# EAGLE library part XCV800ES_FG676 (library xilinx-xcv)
xcv800es_fg676 edit this description Auto generated by make-symbol-device-package-bsdl.ulp Rev. 26 Source: xcv800es_fg676.bsd
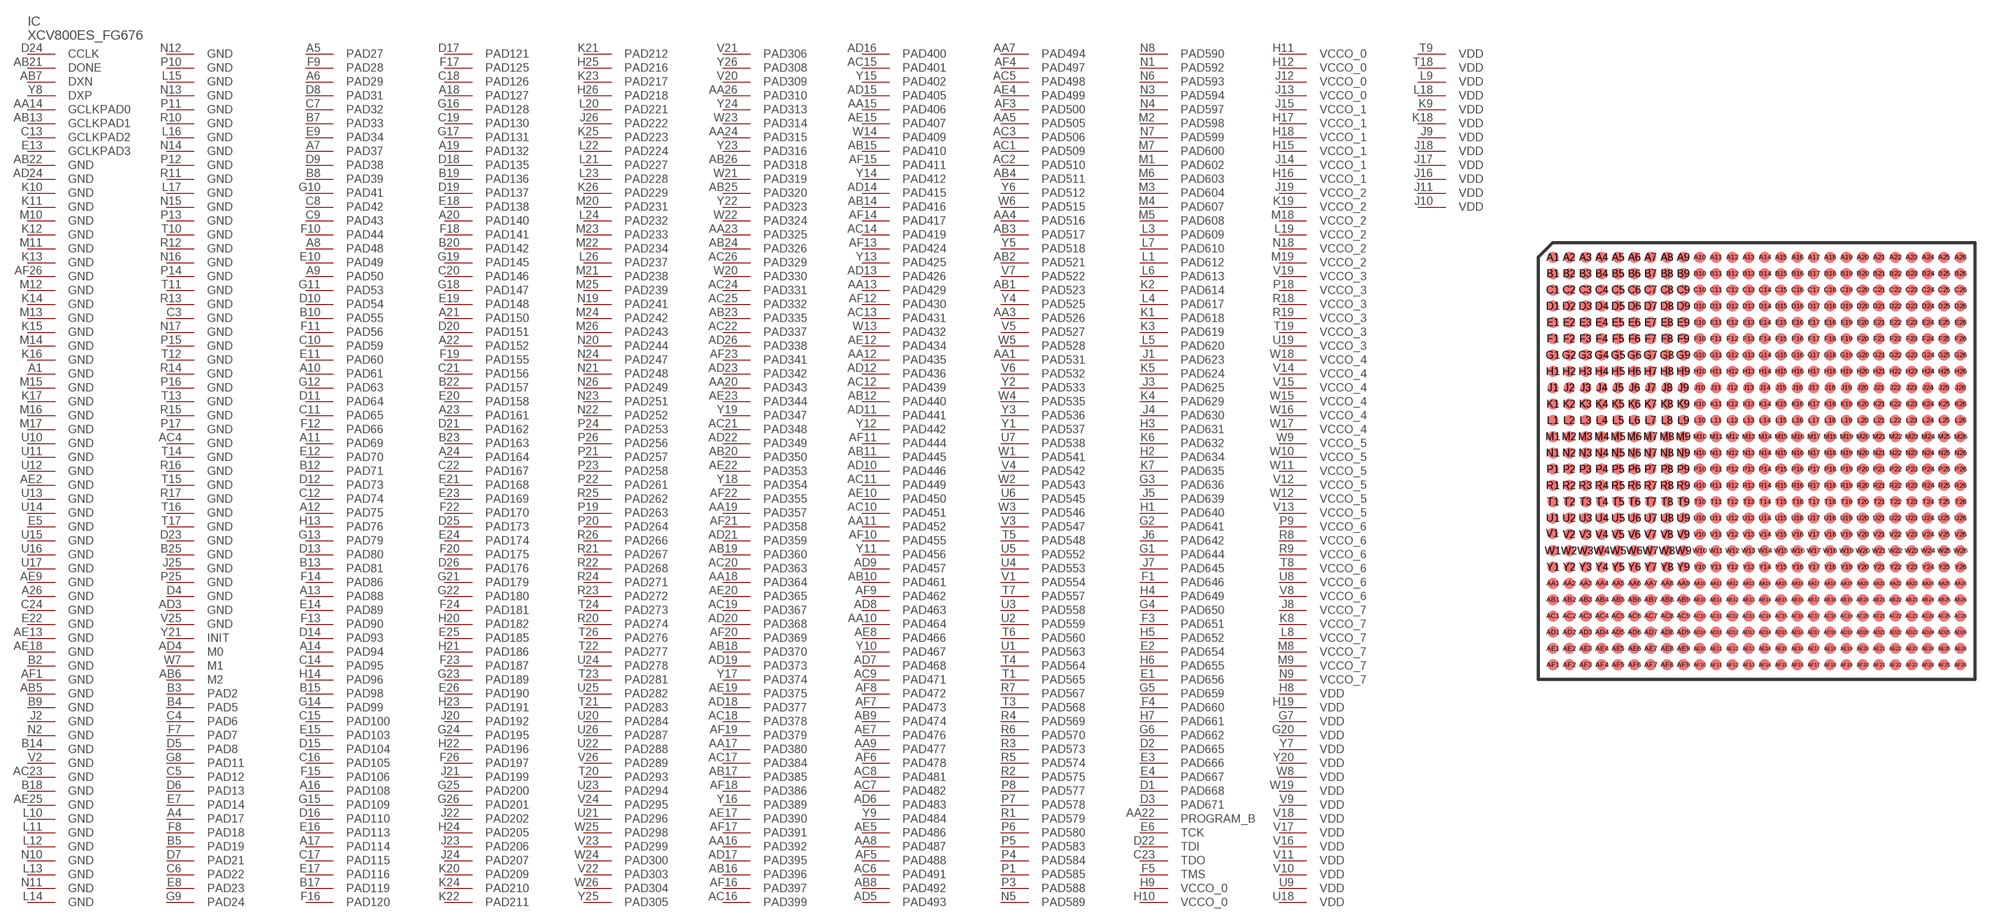
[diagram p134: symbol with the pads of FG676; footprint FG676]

Designator prefix IC

## XCV800ES_FG676 (OC_FARNELL: unknown; OC_NEWARK: unknown)  [FG676]
A1  GND  pwr
A4  PAD17
A5  PAD27
A6  PAD29
A7  PAD37
A8  PAD48
A9  PAD50
A10  PAD61
A11  PAD69
A12  PAD75
A13  PAD88
A14  PAD94
A16  PAD108
A17  PAD114
A18  PAD127
A19  PAD132
A20  PAD140
A21  PAD150
A22  PAD152
A23  PAD161
A24  PAD164
A26  GND  pwr
AA1  PAD531
AA3  PAD526
AA4  PAD516
AA5  PAD505
AA7  PAD494
AA8  PAD487
AA9  PAD477
AA10  PAD464
AA11  PAD452
AA12  PAD435
AA13  PAD429
AA14  GCLKPAD0  in
AA15  PAD406
AA16  PAD392
AA17  PAD380
AA18  PAD364
AA19  PAD357
AA20  PAD343
AA22  PROGRAM_B  in
AA23  PAD325
AA24  PAD315
AA26  PAD310
AB1  PAD523
AB2  PAD521
AB3  PAD517
AB4  PAD511
AB5  GND  pwr
AB6  M2  in
AB7  DXN  pas
AB8  PAD492
AB9  PAD474
AB10  PAD461
AB11  PAD445
AB12  PAD440
AB13  GCLKPAD1  in
AB14  PAD416
AB15  PAD410
AB16  PAD396
AB17  PAD385
AB18  PAD370
AB19  PAD360
AB20  PAD350
AB21  DONE
AB22  GND  pwr
AB23  PAD335
AB24  PAD326
AB25  PAD320
AB26  PAD318
AC1  PAD509
AC2  PAD510
AC3  PAD506
AC4  GND  pwr
AC5  PAD498
AC6  PAD491
AC7  PAD482
AC8  PAD481
AC9  PAD471
AC10  PAD451
AC11  PAD449
AC12  PAD439
AC13  PAD431
AC14  PAD419
AC15  PAD401
AC16  PAD399
AC17  PAD384
AC18  PAD378
AC19  PAD367
AC20  PAD363
AC21  PAD348
AC22  PAD337
AC23  GND  pwr
AC24  PAD331
AC25  PAD332
AC26  PAD329
AD3  GND  pwr
AD4  M0  in
AD5  PAD493
AD6  PAD483
AD7  PAD468
AD8  PAD463
AD9  PAD457
AD10  PAD446
AD11  PAD441
AD12  PAD436
AD13  PAD426
AD14  PAD415
AD15  PAD405
AD16  PAD400
AD17  PAD395
AD18  PAD377
AD19  PAD373
AD20  PAD368
AD21  PAD359
AD22  PAD349
AD23  PAD342
AD24  GND  pwr
AD26  PAD338
AE2  GND  pwr
AE4  PAD499
AE5  PAD486
AE7  PAD476
AE8  PAD466
AE9  GND  pwr
AE10  PAD450
AE12  PAD434
AE13  GND  pwr
AE15  PAD407
AE17  PAD390
AE18  GND  pwr
AE19  PAD375
AE20  PAD365
AE22  PAD353
AE23  PAD344
AE25  GND  pwr
AF1  GND  pwr
AF3  PAD500
AF4  PAD497
AF5  PAD488
AF6  PAD478
AF7  PAD473
AF8  PAD472
AF9  PAD462
AF10  PAD455
AF11  PAD444
AF12  PAD430
AF13  PAD424
AF14  PAD417
AF15  PAD411
AF16  PAD397
AF17  PAD391
AF18  PAD386
AF19  PAD379
AF20  PAD369
AF21  PAD358
AF22  PAD355
AF23  PAD341
AF26  GND  pwr
B2  GND  pwr
B3  PAD2
B4  PAD5
B5  PAD19
B7  PAD33
B8  PAD39
B9  GND  pwr
B10  PAD55
B12  PAD71
B13  PAD81
B14  GND  pwr
B15  PAD98
B17  PAD119
B18  GND  pwr
B19  PAD136
B20  PAD142
B22  PAD157
B23  PAD163
B25  GND  pwr
C3  GND  pwr
C4  PAD6
C5  PAD12
C6  PAD22
C7  PAD32
C8  PAD42
C9  PAD43
C10  PAD59
C11  PAD65
C12  PAD74
C13  GCLKPAD2  in
C14  PAD95
C15  PAD100
C16  PAD105
C17  PAD115
C18  PAD126
C19  PAD130
C20  PAD146
C21  PAD156
C22  PAD167
C23  TDO  out
C24  GND  pwr
D1  PAD668
D2  PAD665
D3  PAD671
D4  GND  pwr
D5  PAD8
D6  PAD13
D7  PAD21
D8  PAD31
D9  PAD38
D10  PAD54
D11  PAD64
D12  PAD73
D13  PAD80
D14  PAD93
D15  PAD104
D16  PAD110
D17  PAD121
D18  PAD135
D19  PAD137
D20  PAD151
D21  PAD162
D22  TDI  in
D23  GND  pwr
D24  CCLK
D25  PAD173
D26  PAD176
E1  PAD656
E2  PAD654
E3  PAD666
E4  PAD667
E5  GND  pwr
E6  TCK  in
E7  PAD14
E8  PAD23
E9  PAD34
E10  PAD49
E11  PAD60
E12  PAD70
E13  GCLKPAD3  in
E14  PAD89
E15  PAD103
E16  PAD113
E17  PAD116
E18  PAD138
E19  PAD148
E20  PAD158
E21  PAD168
E22  GND  pwr
E23  PAD169
E24  PAD174
E25  PAD185
E26  PAD190
F1  PAD646
F3  PAD651
F4  PAD660
F5  TMS  in
F7  PAD7
F8  PAD18
F9  PAD28
F10  PAD44
F11  PAD56
F12  PAD66
F13  PAD90
F14  PAD86
F15  PAD106
F16  PAD120
F17  PAD125
F18  PAD141
F19  PAD155
F20  PAD175
F22  PAD170
F23  PAD187
F24  PAD181
F26  PAD197
G1  PAD644
G2  PAD641
G3  PAD636
G4  PAD650
G5  PAD659
G6  PAD662
G7  VDD  pwr
G8  PAD11
G9  PAD24
G10  PAD41
G11  PAD53
G12  PAD63
G13  PAD79
G14  PAD99
G15  PAD109
G16  PAD128
G17  PAD131
G18  PAD147
G19  PAD145
G20  VDD  pwr
G21  PAD179
G22  PAD180
G23  PAD189
G24  PAD195
G25  PAD200
G26  PAD201
H1  PAD640
H2  PAD634
H3  PAD631
H4  PAD649
H5  PAD652
H6  PAD655
H7  PAD661
H8  VDD  pwr
H9  VCCO_0  pwr
H10  VCCO_0  pwr
H11  VCCO_0  pwr
H12  VCCO_0  pwr
H13  PAD76
H14  PAD96
H15  VCCO_1  pwr
H16  VCCO_1  pwr
H17  VCCO_1  pwr
H18  VCCO_1  pwr
H19  VDD  pwr
H20  PAD182
H21  PAD186
H22  PAD196
H23  PAD191
H24  PAD205
H25  PAD216
H26  PAD218
J1  PAD623
J2  GND  pwr
J3  PAD625
J4  PAD630
J5  PAD639
J6  PAD642
J7  PAD645
J8  VCCO_7  pwr
J9  VDD  pwr
J10  VDD  pwr
J11  VDD  pwr
J12  VCCO_0  pwr
J13  VCCO_0  pwr
J14  VCCO_1  pwr
J15  VCCO_1  pwr
J16  VDD  pwr
J17  VDD  pwr
J18  VDD  pwr
J19  VCCO_2  pwr
J20  PAD192
J21  PAD199
J22  PAD202
J23  PAD206
J24  PAD207
J25  GND  pwr
J26  PAD222
K1  PAD618
K2  PAD614
K3  PAD619
K4  PAD629
K5  PAD624
K6  PAD632
K7  PAD635
K8  VCCO_7  pwr
K9  VDD  pwr
K10  GND  pwr
K11  GND  pwr
K12  GND  pwr
K13  GND  pwr
K14  GND  pwr
K15  GND  pwr
K16  GND  pwr
K17  GND  pwr
K18  VDD  pwr
K19  VCCO_2  pwr
K20  PAD209
K21  PAD212
K22  PAD211
K23  PAD217
K24  PAD210
K25  PAD223
K26  PAD229
L1  PAD612
L3  PAD609
L4  PAD617
L5  PAD620
L6  PAD613
L7  PAD610
L8  VCCO_7  pwr
L9  VDD  pwr
L10  GND  pwr
L11  GND  pwr
L12  GND  pwr
L13  GND  pwr
L14  GND  pwr
L15  GND  pwr
L16  GND  pwr
L17  GND  pwr
L18  VDD  pwr
L19  VCCO_2  pwr
L20  PAD221
L21  PAD227
L22  PAD224
L23  PAD228
L24  PAD232
L26  PAD237
M1  PAD602
M2  PAD598
M3  PAD604
M4  PAD607
M5  PAD608
M6  PAD603
M7  PAD600
M8  VCCO_7  pwr
M9  VCCO_7  pwr
M10  GND  pwr
M11  GND  pwr
M12  GND  pwr
M13  GND  pwr
M14  GND  pwr
M15  GND  pwr
M16  GND  pwr
M17  GND  pwr
M18  VCCO_2  pwr
M19  VCCO_2  pwr
M20  PAD231
M21  PAD238
M22  PAD234
M23  PAD233
M24  PAD242
M25  PAD239
M26  PAD243
N1  PAD592
N2  GND  pwr
N3  PAD594
N4  PAD597
N5  PAD589
N6  PAD593
N7  PAD599
N8  PAD590
N9  VCCO_7  pwr
N10  GND  pwr
N11  GND  pwr
N12  GND  pwr
N13  GND  pwr
N14  GND  pwr
N15  GND  pwr
N16  GND  pwr
N17  GND  pwr
N18  VCCO_2  pwr
N19  PAD241
N20  PAD244
N21  PAD248
N22  PAD252
N23  PAD251
N24  PAD247
N26  PAD249
P1  PAD585
P3  PAD588
P4  PAD584
P5  PAD583
P6  PAD580
P7  PAD578
P8  PAD577
P9  VCCO_6  pwr
P10  GND  pwr
P11  GND  pwr
P12  GND  pwr
P13  GND  pwr
P14  GND  pwr
P15  GND  pwr
P16  GND  pwr
P17  GND  pwr
P18  VCCO_3  pwr
P19  PAD263
P20  PAD264
P21  PAD257
P22  PAD261
P23  PAD258
P24  PAD253
P25  GND  pwr
P26  PAD256
R1  PAD579
R2  PAD575
R3  PAD573
R4  PAD569
R5  PAD574
R6  PAD570
R7  PAD567
R8  VCCO_6  pwr
R9  VCCO_6  pwr
R10  GND  pwr
R11  GND  pwr
R12  GND  pwr
R13  GND  pwr
R14  GND  pwr
R15  GND  pwr
R16  GND  pwr
R17  GND  pwr
R18  VCCO_3  pwr
R19  VCCO_3  pwr
R20  PAD274
R21  PAD267
R22  PAD268
R23  PAD272
R24  PAD271
R25  PAD262
R26  PAD266
T1  PAD565
T3  PAD568
T4  PAD564
T5  PAD548
T6  PAD560
T7  PAD557
T8  VCCO_6  pwr
T9  VDD  pwr
T10  GND  pwr
T11  GND  pwr
T12  GND  pwr
T13  GND  pwr
T14  GND  pwr
T15  GND  pwr
T16  GND  pwr
T17  GND  pwr
T18  VDD  pwr
T19  VCCO_3  pwr
T20  PAD293
T21  PAD283
T22  PAD277
T23  PAD281
T24  PAD273
T26  PAD276
U1  PAD563
U2  PAD559
U3  PAD558
U4  PAD553
U5  PAD552
U6  PAD545
U7  PAD538
U8  VCCO_6  pwr
U9  VDD  pwr
U10  GND  pwr
U11  GND  pwr
U12  GND  pwr
U13  GND  pwr
U14  GND  pwr
U15  GND  pwr
U16  GND  pwr
U17  GND  pwr
U18  VDD  pwr
U19  VCCO_3  pwr
U20  PAD284
U21  PAD296
U22  PAD288
U23  PAD294
U24  PAD278
U25  PAD282
U26  PAD287
V1  PAD554
V2  GND  pwr
V3  PAD547
V4  PAD542
V5  PAD527
V6  PAD532
V7  PAD522
V8  VCCO_6  pwr
V9  VDD  pwr
V10  VDD  pwr
V11  VDD  pwr
V12  VCCO_5  pwr
V13  VCCO_5  pwr
V14  VCCO_4  pwr
V15  VCCO_4  pwr
V16  VDD  pwr
V17  VDD  pwr
V18  VDD  pwr
V19  VCCO_3  pwr
V20  PAD309
V21  PAD306
V22  PAD303
V23  PAD299
V24  PAD295
V25  GND  pwr
V26  PAD289
W1  PAD541
W2  PAD543
W3  PAD546
W4  PAD535
W5  PAD528
W6  PAD515
W7  M1  in
W8  VDD  pwr
W9  VCCO_5  pwr
W10  VCCO_5  pwr
W11  VCCO_5  pwr
W12  VCCO_5  pwr
W13  PAD432
W14  PAD409
W15  VCCO_4  pwr
W16  VCCO_4  pwr
W17  VCCO_4  pwr
W18  VCCO_4  pwr
W19  VDD  pwr
W20  PAD330
W21  PAD319
W22  PAD324
W23  PAD314
W24  PAD300
W25  PAD298
W26  PAD304
Y1  PAD537
Y2  PAD533
Y3  PAD536
Y4  PAD525
Y5  PAD518
Y6  PAD512
Y7  VDD  pwr
Y8  DXP  pas
Y9  PAD484
Y10  PAD467
Y11  PAD456
Y12  PAD442
Y13  PAD425
Y14  PAD412
Y15  PAD402
Y16  PAD389
Y17  PAD374
Y18  PAD354
Y19  PAD347
Y20  VDD  pwr
Y21  INIT
Y22  PAD323
Y23  PAD316
Y24  PAD313
Y25  PAD305
Y26  PAD308

## Footprint FG676 (pad centres in mm)
xcv400_fg676 edit this description Auto generated by make-symbol-device-package-bsdl.ulp Rev. 26 Source: xcv400_fg676.bsd
smd 0.7 x 0.7: A1 -12.5,12.5; A2 -11.5,12.5; A3 -10.5,12.5; A4 -9.5,12.5; A5 -8.5,12.5; A6 -7.5,12.5; A7 -6.5,12.5; A8 -5.5,12.5; A9 -4.5,12.5; A10 -3.5,12.5; A11 -2.5,12.5; A12 -1.5,12.5; A13 -0.5,12.5; A14 0.5,12.5; A15 1.5,12.5; A16 2.5,12.5; A17 3.5,12.5; A18 4.5,12.5; A19 5.5,12.5; A20 6.5,12.5; A21 7.5,12.5; A22 8.5,12.5; A23 9.5,12.5; A24 10.5,12.5; A25 11.5,12.5; A26 12.5,12.5; AA1 -12.5,-7.5; AA2 -11.5,-7.5; AA3 -10.5,-7.5; AA4 -9.5,-7.5; AA5 -8.5,-7.5; AA6 -7.5,-7.5; AA7 -6.5,-7.5; AA8 -5.5,-7.5; AA9 -4.5,-7.5; AA10 -3.5,-7.5; AA11 -2.5,-7.5; AA12 -1.5,-7.5; AA13 -0.5,-7.5; AA14 0.5,-7.5; AA15 1.5,-7.5; AA16 2.5,-7.5; AA17 3.5,-7.5; AA18 4.5,-7.5; AA19 5.5,-7.5; AA20 6.5,-7.5; AA21 7.5,-7.5; AA22 8.5,-7.5; AA23 9.5,-7.5; AA24 10.5,-7.5; AA25 11.5,-7.5; AA26 12.5,-7.5; AB1 -12.5,-8.5; AB2 -11.5,-8.5; AB3 -10.5,-8.5; AB4 -9.5,-8.5; AB5 -8.5,-8.5; AB6 -7.5,-8.5; AB7 -6.5,-8.5; AB8 -5.5,-8.5; AB9 -4.5,-8.5; AB10 -3.5,-8.5; AB11 -2.5,-8.5; AB12 -1.5,-8.5; AB13 -0.5,-8.5; AB14 0.5,-8.5; AB15 1.5,-8.5; AB16 2.5,-8.5; AB17 3.5,-8.5; AB18 4.5,-8.5; AB19 5.5,-8.5; AB20 6.5,-8.5; AB21 7.5,-8.5; AB22 8.5,-8.5; AB23 9.5,-8.5; AB24 10.5,-8.5; AB25 11.5,-8.5; AB26 12.5,-8.5; AC1 -12.5,-9.5; AC2 -11.5,-9.5; AC3 -10.5,-9.5; AC4 -9.5,-9.5; AC5 -8.5,-9.5; AC6 -7.5,-9.5; AC7 -6.5,-9.5; AC8 -5.5,-9.5; AC9 -4.5,-9.5; AC10 -3.5,-9.5; AC11 -2.5,-9.5; AC12 -1.5,-9.5; AC13 -0.5,-9.5; AC14 0.5,-9.5; AC15 1.5,-9.5; AC16 2.5,-9.5; AC17 3.5,-9.5; AC18 4.5,-9.5; AC19 5.5,-9.5; AC20 6.5,-9.5; AC21 7.5,-9.5; AC22 8.5,-9.5; AC23 9.5,-9.5; AC24 10.5,-9.5; AC25 11.5,-9.5; AC26 12.5,-9.5; AD1 -12.5,-10.5; AD2 -11.5,-10.5; AD3 -10.5,-10.5; AD4 -9.5,-10.5; AD5 -8.5,-10.5; AD6 -7.5,-10.5; AD7 -6.5,-10.5; AD8 -5.5,-10.5; AD9 -4.5,-10.5; AD10 -3.5,-10.5; AD11 -2.5,-10.5; AD12 -1.5,-10.5; AD13 -0.5,-10.5; AD14 0.5,-10.5; AD15 1.5,-10.5; AD16 2.5,-10.5; AD17 3.5,-10.5; AD18 4.5,-10.5; AD19 5.5,-10.5; AD20 6.5,-10.5; AD21 7.5,-10.5; AD22 8.5,-10.5; AD23 9.5,-10.5; AD24 10.5,-10.5; AD25 11.5,-10.5; AD26 12.5,-10.5; AE1 -12.5,-11.5; AE2 -11.5,-11.5; AE3 -10.5,-11.5; AE4 -9.5,-11.5; AE5 -8.5,-11.5; AE6 -7.5,-11.5; AE7 -6.5,-11.5; AE8 -5.5,-11.5; AE9 -4.5,-11.5; AE10 -3.5,-11.5; AE11 -2.5,-11.5; AE12 -1.5,-11.5; AE13 -0.5,-11.5; AE14 0.5,-11.5; AE15 1.5,-11.5; AE16 2.5,-11.5; AE17 3.5,-11.5; AE18 4.5,-11.5; AE19 5.5,-11.5; AE20 6.5,-11.5; AE21 7.5,-11.5; AE22 8.5,-11.5; AE23 9.5,-11.5; AE24 10.5,-11.5; AE25 11.5,-11.5; AE26 12.5,-11.5; AF1 -12.5,-12.5; AF2 -11.5,-12.5; AF3 -10.5,-12.5; AF4 -9.5,-12.5; AF5 -8.5,-12.5; AF6 -7.5,-12.5; AF7 -6.5,-12.5; AF8 -5.5,-12.5; AF9 -4.5,-12.5; AF10 -3.5,-12.5; AF11 -2.5,-12.5; AF12 -1.5,-12.5; AF13 -0.5,-12.5; AF14 0.5,-12.5; AF15 1.5,-12.5; AF16 2.5,-12.5; AF17 3.5,-12.5; AF18 4.5,-12.5; AF19 5.5,-12.5; AF20 6.5,-12.5; AF21 7.5,-12.5; AF22 8.5,-12.5; AF23 9.5,-12.5; AF24 10.5,-12.5; AF25 11.5,-12.5; AF26 12.5,-12.5; B1 -12.5,11.5; B2 -11.5,11.5; B3 -10.5,11.5; B4 -9.5,11.5; B5 -8.5,11.5; B6 -7.5,11.5; B7 -6.5,11.5; B8 -5.5,11.5; B9 -4.5,11.5; B10 -3.5,11.5; B11 -2.5,11.5; B12 -1.5,11.5; B13 -0.5,11.5; B14 0.5,11.5; B15 1.5,11.5; B16 2.5,11.5; B17 3.5,11.5; B18 4.5,11.5; B19 5.5,11.5; B20 6.5,11.5; B21 7.5,11.5; B22 8.5,11.5; B23 9.5,11.5; B24 10.5,11.5; B25 11.5,11.5; B26 12.5,11.5; C1 -12.5,10.5; C2 -11.5,10.5; C3 -10.5,10.5; C4 -9.5,10.5; C5 -8.5,10.5; C6 -7.5,10.5; C7 -6.5,10.5; C8 -5.5,10.5; C9 -4.5,10.5; C10 -3.5,10.5; C11 -2.5,10.5; C12 -1.5,10.5; C13 -0.5,10.5; C14 0.5,10.5; C15 1.5,10.5; C16 2.5,10.5; C17 3.5,10.5; C18 4.5,10.5; C19 5.5,10.5; C20 6.5,10.5; C21 7.5,10.5; C22 8.5,10.5; C23 9.5,10.5; C24 10.5,10.5; C25 11.5,10.5; C26 12.5,10.5; D1 -12.5,9.5; D2 -11.5,9.5; D3 -10.5,9.5; D4 -9.5,9.5; D5 -8.5,9.5; D6 -7.5,9.5; D7 -6.5,9.5; D8 -5.5,9.5; D9 -4.5,9.5; D10 -3.5,9.5; D11 -2.5,9.5; D12 -1.5,9.5; D13 -0.5,9.5; D14 0.5,9.5; D15 1.5,9.5; D16 2.5,9.5; D17 3.5,9.5; D18 4.5,9.5; D19 5.5,9.5; D20 6.5,9.5; D21 7.5,9.5; D22 8.5,9.5; D23 9.5,9.5; D24 10.5,9.5; D25 11.5,9.5; D26 12.5,9.5; E1 -12.5,8.5; E2 -11.5,8.5; E3 -10.5,8.5; E4 -9.5,8.5; E5 -8.5,8.5; E6 -7.5,8.5; E7 -6.5,8.5; E8 -5.5,8.5; E9 -4.5,8.5; E10 -3.5,8.5; E11 -2.5,8.5; E12 -1.5,8.5; E13 -0.5,8.5; E14 0.5,8.5; E15 1.5,8.5; E16 2.5,8.5; E17 3.5,8.5; E18 4.5,8.5; E19 5.5,8.5; E20 6.5,8.5; E21 7.5,8.5; E22 8.5,8.5; E23 9.5,8.5; E24 10.5,8.5; E25 11.5,8.5; E26 12.5,8.5; F1 -12.5,7.5; F2 -11.5,7.5; F3 -10.5,7.5; F4 -9.5,7.5; F5 -8.5,7.5; F6 -7.5,7.5; F7 -6.5,7.5; F8 -5.5,7.5; F9 -4.5,7.5; F10 -3.5,7.5; F11 -2.5,7.5; F12 -1.5,7.5; F13 -0.5,7.5; F14 0.5,7.5; F15 1.5,7.5; F16 2.5,7.5; F17 3.5,7.5; F18 4.5,7.5; F19 5.5,7.5; F20 6.5,7.5; F21 7.5,7.5; F22 8.5,7.5; F23 9.5,7.5; F24 10.5,7.5; F25 11.5,7.5; F26 12.5,7.5; G1 -12.5,6.5; G2 -11.5,6.5; G3 -10.5,6.5; G4 -9.5,6.5; G5 -8.5,6.5; G6 -7.5,6.5; G7 -6.5,6.5; G8 -5.5,6.5; G9 -4.5,6.5; G10 -3.5,6.5; G11 -2.5,6.5; G12 -1.5,6.5; G13 -0.5,6.5; G14 0.5,6.5; G15 1.5,6.5; G16 2.5,6.5; G17 3.5,6.5; G18 4.5,6.5; G19 5.5,6.5; G20 6.5,6.5; G21 7.5,6.5; G22 8.5,6.5; G23 9.5,6.5; G24 10.5,6.5; G25 11.5,6.5; G26 12.5,6.5; H1 -12.5,5.5; H2 -11.5,5.5; H3 -10.5,5.5; H4 -9.5,5.5; H5 -8.5,5.5; H6 -7.5,5.5; H7 -6.5,5.5; H8 -5.5,5.5; H9 -4.5,5.5; H10 -3.5,5.5; H11 -2.5,5.5; H12 -1.5,5.5; H13 -0.5,5.5; H14 0.5,5.5; H15 1.5,5.5; H16 2.5,5.5; H17 3.5,5.5; H18 4.5,5.5; H19 5.5,5.5; H20 6.5,5.5; H21 7.5,5.5; H22 8.5,5.5; H23 9.5,5.5; H24 10.5,5.5; H25 11.5,5.5; H26 12.5,5.5; J1 -12.5,4.5; J2 -11.5,4.5; J3 -10.5,4.5; J4 -9.5,4.5; J5 -8.5,4.5; J6 -7.5,4.5; J7 -6.5,4.5; J8 -5.5,4.5; J9 -4.5,4.5; J10 -3.5,4.5; J11 -2.5,4.5; J12 -1.5,4.5; J13 -0.5,4.5; J14 0.5,4.5; J15 1.5,4.5; J16 2.5,4.5; J17 3.5,4.5; J18 4.5,4.5; J19 5.5,4.5; J20 6.5,4.5; J21 7.5,4.5; J22 8.5,4.5; J23 9.5,4.5; J24 10.5,4.5; J25 11.5,4.5; J26 12.5,4.5; K1 -12.5,3.5; K2 -11.5,3.5; K3 -10.5,3.5; K4 -9.5,3.5; K5 -8.5,3.5; K6 -7.5,3.5; K7 -6.5,3.5; K8 -5.5,3.5; K9 -4.5,3.5; K10 -3.5,3.5; K11 -2.5,3.5; K12 -1.5,3.5; K13 -0.5,3.5; K14 0.5,3.5; K15 1.5,3.5; K16 2.5,3.5; K17 3.5,3.5; K18 4.5,3.5; K19 5.5,3.5; K20 6.5,3.5; K21 7.5,3.5; K22 8.5,3.5; K23 9.5,3.5; K24 10.5,3.5; K25 11.5,3.5; K26 12.5,3.5; L1 -12.5,2.5; L2 -11.5,2.5; L3 -10.5,2.5; L4 -9.5,2.5; L5 -8.5,2.5; L6 -7.5,2.5; L7 -6.5,2.5; L8 -5.5,2.5; L9 -4.5,2.5; L10 -3.5,2.5; L11 -2.5,2.5; L12 -1.5,2.5; L13 -0.5,2.5; L14 0.5,2.5; L15 1.5,2.5; L16 2.5,2.5; L17 3.5,2.5; L18 4.5,2.5; L19 5.5,2.5; L20 6.5,2.5; L21 7.5,2.5; L22 8.5,2.5; L23 9.5,2.5; L24 10.5,2.5; L25 11.5,2.5; L26 12.5,2.5; M1 -12.5,1.5; M2 -11.5,1.5; M3 -10.5,1.5; M4 -9.5,1.5; M5 -8.5,1.5; M6 -7.5,1.5; M7 -6.5,1.5; M8 -5.5,1.5; M9 -4.5,1.5; M10 -3.5,1.5; M11 -2.5,1.5; M12 -1.5,1.5; M13 -0.5,1.5; M14 0.5,1.5; M15 1.5,1.5; M16 2.5,1.5; M17 3.5,1.5; M18 4.5,1.5; M19 5.5,1.5; M20 6.5,1.5; M21 7.5,1.5; M22 8.5,1.5; M23 9.5,1.5; M24 10.5,1.5; M25 11.5,1.5; M26 12.5,1.5; N1 -12.5,0.5; N2 -11.5,0.5; N3 -10.5,0.5; N4 -9.5,0.5; N5 -8.5,0.5; N6 -7.5,0.5; N7 -6.5,0.5; N8 -5.5,0.5; N9 -4.5,0.5; N10 -3.5,0.5; N11 -2.5,0.5; N12 -1.5,0.5; N13 -0.5,0.5; N14 0.5,0.5; N15 1.5,0.5; N16 2.5,0.5; N17 3.5,0.5; N18 4.5,0.5; N19 5.5,0.5; N20 6.5,0.5; N21 7.5,0.5; N22 8.5,0.5; N23 9.5,0.5; N24 10.5,0.5; N25 11.5,0.5; N26 12.5,0.5; P1 -12.5,-0.5; P2 -11.5,-0.5; P3 -10.5,-0.5; P4 -9.5,-0.5; P5 -8.5,-0.5; P6 -7.5,-0.5; P7 -6.5,-0.5; P8 -5.5,-0.5; P9 -4.5,-0.5; P10 -3.5,-0.5; P11 -2.5,-0.5; P12 -1.5,-0.5; P13 -0.5,-0.5; P14 0.5,-0.5; P15 1.5,-0.5; P16 2.5,-0.5; P17 3.5,-0.5; P18 4.5,-0.5; P19 5.5,-0.5; P20 6.5,-0.5; P21 7.5,-0.5; P22 8.5,-0.5; P23 9.5,-0.5; P24 10.5,-0.5; P25 11.5,-0.5; P26 12.5,-0.5; R1 -12.5,-1.5; R2 -11.5,-1.5; R3 -10.5,-1.5; R4 -9.5,-1.5; R5 -8.5,-1.5; R6 -7.5,-1.5; R7 -6.5,-1.5; R8 -5.5,-1.5; R9 -4.5,-1.5; R10 -3.5,-1.5; R11 -2.5,-1.5; R12 -1.5,-1.5; R13 -0.5,-1.5; R14 0.5,-1.5; R15 1.5,-1.5; R16 2.5,-1.5; R17 3.5,-1.5; R18 4.5,-1.5; R19 5.5,-1.5; R20 6.5,-1.5; R21 7.5,-1.5; R22 8.5,-1.5; R23 9.5,-1.5; R24 10.5,-1.5; R25 11.5,-1.5; R26 12.5,-1.5; T1 -12.5,-2.5; T2 -11.5,-2.5; T3 -10.5,-2.5; T4 -9.5,-2.5; T5 -8.5,-2.5; T6 -7.5,-2.5; T7 -6.5,-2.5; T8 -5.5,-2.5; T9 -4.5,-2.5; T10 -3.5,-2.5; T11 -2.5,-2.5; T12 -1.5,-2.5; T13 -0.5,-2.5; T14 0.5,-2.5; T15 1.5,-2.5; T16 2.5,-2.5; T17 3.5,-2.5; T18 4.5,-2.5; T19 5.5,-2.5; T20 6.5,-2.5; T21 7.5,-2.5; T22 8.5,-2.5; T23 9.5,-2.5; T24 10.5,-2.5; T25 11.5,-2.5; T26 12.5,-2.5; U1 -12.5,-3.5; U2 -11.5,-3.5; U3 -10.5,-3.5; U4 -9.5,-3.5; U5 -8.5,-3.5; U6 -7.5,-3.5; U7 -6.5,-3.5; U8 -5.5,-3.5; U9 -4.5,-3.5; U10 -3.5,-3.5; U11 -2.5,-3.5; U12 -1.5,-3.5; U13 -0.5,-3.5; U14 0.5,-3.5; U15 1.5,-3.5; U16 2.5,-3.5; U17 3.5,-3.5; U18 4.5,-3.5; U19 5.5,-3.5; U20 6.5,-3.5; U21 7.5,-3.5; U22 8.5,-3.5; U23 9.5,-3.5; U24 10.5,-3.5; U25 11.5,-3.5; U26 12.5,-3.5; V1 -12.527,-4.431; V2 -11.5,-4.5; V3 -10.5,-4.5; V4 -9.5,-4.5; V5 -8.5,-4.5; V6 -7.5,-4.5; V7 -6.5,-4.5; V8 -5.5,-4.5; V9 -4.5,-4.5; V10 -3.5,-4.5; V11 -2.5,-4.5; V12 -1.5,-4.5; V13 -0.5,-4.5; V14 0.5,-4.5; V15 1.5,-4.5; V16 2.5,-4.5; V17 3.5,-4.5; V18 4.5,-4.5; V19 5.5,-4.5; V20 6.5,-4.5; V21 7.5,-4.5; V22 8.5,-4.5; V23 9.5,-4.5; V24 10.5,-4.5; V25 11.5,-4.5; V26 12.5,-4.5; W1 -12.5,-5.5; W2 -11.5,-5.5; W3 -10.5,-5.5; W4 -9.5,-5.5; W5 -8.5,-5.5; W6 -7.5,-5.5; W7 -6.5,-5.5; W8 -5.5,-5.5; W9 -4.5,-5.5; W10 -3.5,-5.5; W11 -2.5,-5.5; W12 -1.5,-5.5; W13 -0.5,-5.5; W14 0.5,-5.5; W15 1.5,-5.5; W16 2.5,-5.5; W17 3.5,-5.5; W18 4.5,-5.5; W19 5.5,-5.5; W20 6.5,-5.5; W21 7.5,-5.5; W22 8.5,-5.5; W23 9.5,-5.5; W24 10.5,-5.5; W25 11.5,-5.5; W26 12.5,-5.5; Y1 -12.5,-6.5; Y2 -11.5,-6.5; Y3 -10.5,-6.5; Y4 -9.5,-6.5; Y5 -8.5,-6.5; Y6 -7.5,-6.5; Y7 -6.5,-6.5; Y8 -5.5,-6.5; Y9 -4.5,-6.5; Y10 -3.5,-6.5; Y11 -2.5,-6.5; Y12 -1.5,-6.5; Y13 -0.5,-6.5; Y14 0.5,-6.5; Y15 1.5,-6.5; Y16 2.5,-6.5; Y17 3.5,-6.5; Y18 4.5,-6.5; Y19 5.5,-6.5; Y20 6.5,-6.5; Y21 7.5,-6.5; Y22 8.5,-6.5; Y23 9.5,-6.5; Y24 10.5,-6.5; Y25 11.5,-6.5; Y26 12.5,-6.5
